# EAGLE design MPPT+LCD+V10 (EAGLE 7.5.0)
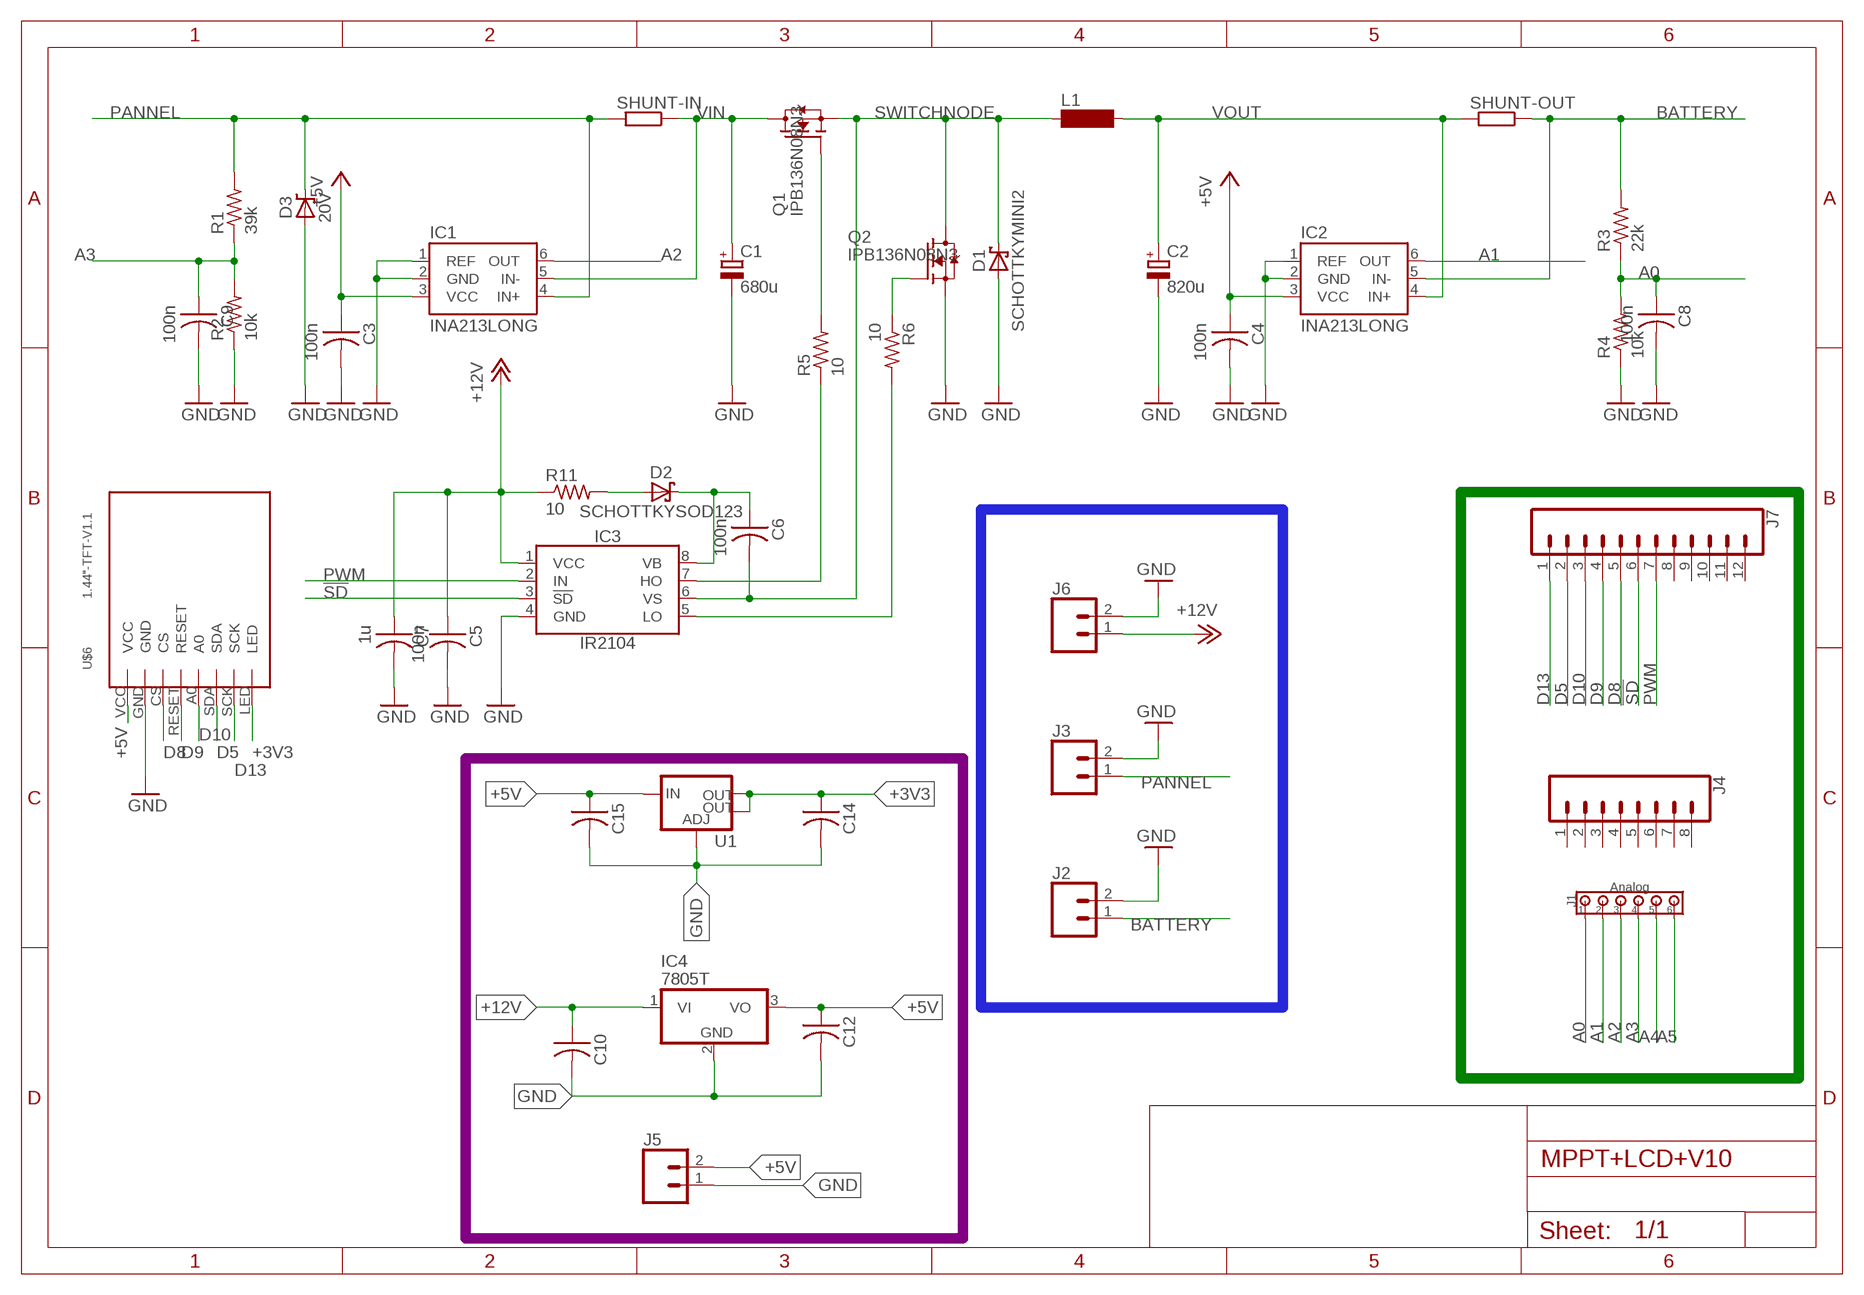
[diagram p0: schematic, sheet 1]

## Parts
C1  680u  C_POLARIZED10MM  [10MM]
C2  820u  C_POLARIZED10MM  [10MM]
C3  100n  CAP-US1206FAB  [C1206FAB]
C4  100n  CAP-US1206FAB  [C1206FAB]
C5  100n  CAP-US1206FAB  [C1206FAB]
C6  100n  CAP-US1206FAB  [C1206FAB]
C7  1u  CAP-US1206FAB  [C1206FAB]
C8  100n  CAP-US1206FAB  [C1206FAB]
C9  100n  CAP-US1206FAB  [C1206FAB]
C10  CAP-US1206FAB  [C1206FAB]
C12  CAP-US1206FAB  [C1206FAB]
C14  CAP-US1206FAB  [C1206FAB]
C15  CAP-US1206FAB  [C1206FAB]
D1  SCHOTTKYMINI2  [MINI2-F3-B]
D2  SCHOTTKYSOD123  [SOD123]
D3  20V  ZENERSMC  [SMC]
IC1  INA213LONG  [SC70-6_LONG]
IC2  INA213LONG  [SC70-6_LONG]
IC3  IR2104  [SOIC8]
IC4  7805T  [TO220H]
J1  Analog  100MIL_6X  [100MIL_6X_ROUND]
J2  CONN_02PTH4  [1X02_XTRA_BIG]
J3  CONN_02PTH4  [1X02_XTRA_BIG]
J4  CONN_08"  [1X08]
J5  CONN_02  [1X02]
J6  CONN_02PTH4  [1X02_XTRA_BIG]
J7  CONN_12  [1X12]
L1  SD75  [SD75]
Q1  IPB136N08N3  N-PWR-MOSFETTO263-3  [TO263-3]
Q2  IPB136N08N3  IPB136N08N3_GTO263  [TO263-3@1]
R1  39k  RES-US1206FAB  [R1206FAB]
R2  10k  RES-US1206FAB  [R1206FAB]
R3  22k  RES-US1206FAB  [R1206FAB]
R4  10k  RES-US1206FAB  [R1206FAB]
R5  10  RES-US1206FAB  [R1206FAB]
R6  10  RES-US1206FAB  [R1206FAB]
R11  10  RES-US1206FAB  [R1206FAB]
SHUNT-IN  SMR  [SMR]
SHUNT-OUT  SMR  [SMR]
U1  V_REG_LM1117SOT223  [SOT223]
U$6  1.44"-TFT-V1.1  [1.44-TFT-V1.1]

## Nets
!SD!: IC3.3(!SD!) J7.6
+3V3: C14.1 U1.2(OUT) U1.4(OUT) U$6.LED
+5V: C3.1 C4.1 C12.1 C15.1 IC1.3(VCC) IC2.3(VCC) IC4.3(VO) J5.2 U1.3(IN) U$6.VCC
+12V: C5.1 C7.1 C10.1 IC3.1(VCC) IC4.1(VI) J6.1 R11.1
A0: C8.1 J1.1 R3.1 R4.2
A1: IC2.6(OUT) J1.2
A2: IC1.6(OUT) J1.3
A3: C9.1 J1.4 R1.1 R2.2
A4: J1.5
A5: J1.6
BATTERY: IC2.5(IN-) J2.1 R3.2 SHUNT-OUT.1
D5: J7.2 U$6.SDA
D8: J7.5 U$6.CS
D9: J7.4 U$6.RESET
D10: J7.3 U$6.A0
D13: J7.1 U$6.SCK
GND: C1.- C2.- C3.2 C4.2 C5.2 C7.2 C8.2 C9.2 C10.2 C12.2 C14.2 C15.2 D1.A D3.A IC1.1(REF) IC1.2(GND) IC2.1(REF) IC2.2(GND) IC3.4(GND) IC4.2(GND) J2.2 J3.2 J5.1 J6.2 Q2.3(S) R2.1 R4.1 U1.1(ADJ) U$6.GND
N$4: Q1.1(G) R5.2
N$7: Q2.1(G) R6.1
N$11: D2.A R11.2
N$12: C6.1 D2.C IC3.8(VB)
N$14: IC3.7(HO) R5.1
N$15: IC3.5(LO) R6.2
PANNEL: D3.C IC1.4(IN+) J3.1 R1.2 SHUNT-IN.2
PWM: IC3.2(IN) J7.7
SWITCHNODE: C6.2 D1.C IC3.6(VS) L1.1 Q1.3(S) Q2.TAB(D)
VIN: C1.+ IC1.5(IN-) Q1.TAB(D) SHUNT-IN.1
VOUT: C2.+ IC2.4(IN+) L1.2 SHUNT-OUT.2
Unconnected: J4.1 J4.2 J4.3 J4.4 J4.5 J4.6 J4.7 J4.8 J7.8 J7.9 J7.10 J7.11 J7.12

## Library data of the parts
C1 C2 = 00Capacitor:C_POLARIZED
C3-C10 C12 C14 C15 = fab:CAP-US
D1 D2 = 00Diode:SCHOTTKY
D3 = 00Diode:ZENER
IC1 IC2 = 00Sensor:INA21*: Current-Shunt Monitors Voltage Output, Low- or High-Side Measurement, Bidirectional, Zero-Drift Series; GAIN: 50
IC3 = 00Logic:IR2104: Half-Bridge Driver Up to +600V Gate drive supply 10-20V Deadtime 520ns
IC4 = linear:78*: Positive VOLTAGE REGULATOR Source: http://cache.national.com/ds/LM/LM78L05.pdf http://www.fairchildsemi.com/ds/LM/LM7805.pdf
J1 = 00Connector:100MIL_6X: 100 mil 6-pin connector
J2 J3 J5 J6 = SparkFun-Connectors:CONN_02: Multi connection point. Often used as Generic Header-pin footprint for 0.1 inch spaced/style header connections
J4 = SparkFun-Connectors:CONN_08: Multi connection point. Often used as Generic Header-pin footprint for 0.1 inch spaced/style header connections On any of the 0.1 inch spaced packages, you can populate with these: Break Away Headers - Straight (PRT-00116) Break Away Male Headers - Right Angle (PRT-00553) Female Headers (PRT-00115)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; PROD_ID: CONN-08438
J7 = SparkFun-Connectors:CONN_12: Multi connection point. Often used as Generic Header-pin footprint for 0.1 inch spaced/style header connections On any of the 0.1 inch spaced packages, you can populate with these: Break Away Headers - Straight (PRT-00116) Break Away Male Headers - Right Angle (PRT-00553) Female Headers (PRT-00115)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
L1 = inductor-neosid:SD75: INDUCTOR; OC_FARNELL: unknown; OC_NEWARK: unknown
Q1 = 00Mosfet:N-PWR-MOSFET
Q2 = 00Mosfet:IPB136N08N3_G
R1-R6 R11 = fab:RES-US: Resistor (US Symbol)
SHUNT-IN SHUNT-OUT = resistor-shunt:SMR: SMD SHUNT RESISTOR; OC_FARNELL: unknown; OC_NEWARK: unknown
U1 = fab:V_REG_LM1117: Voltage Regulator LM1117 Standard adjustable voltage regulator but in SMD form. Spark Fun Electronics SKU : COM-00595; PROD_ID: VREG-08170
U$6 = tft_1.8_1.44_oled_0.96:1.44"-TFT-V1.1

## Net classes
0 default: clearance 0.205 mm

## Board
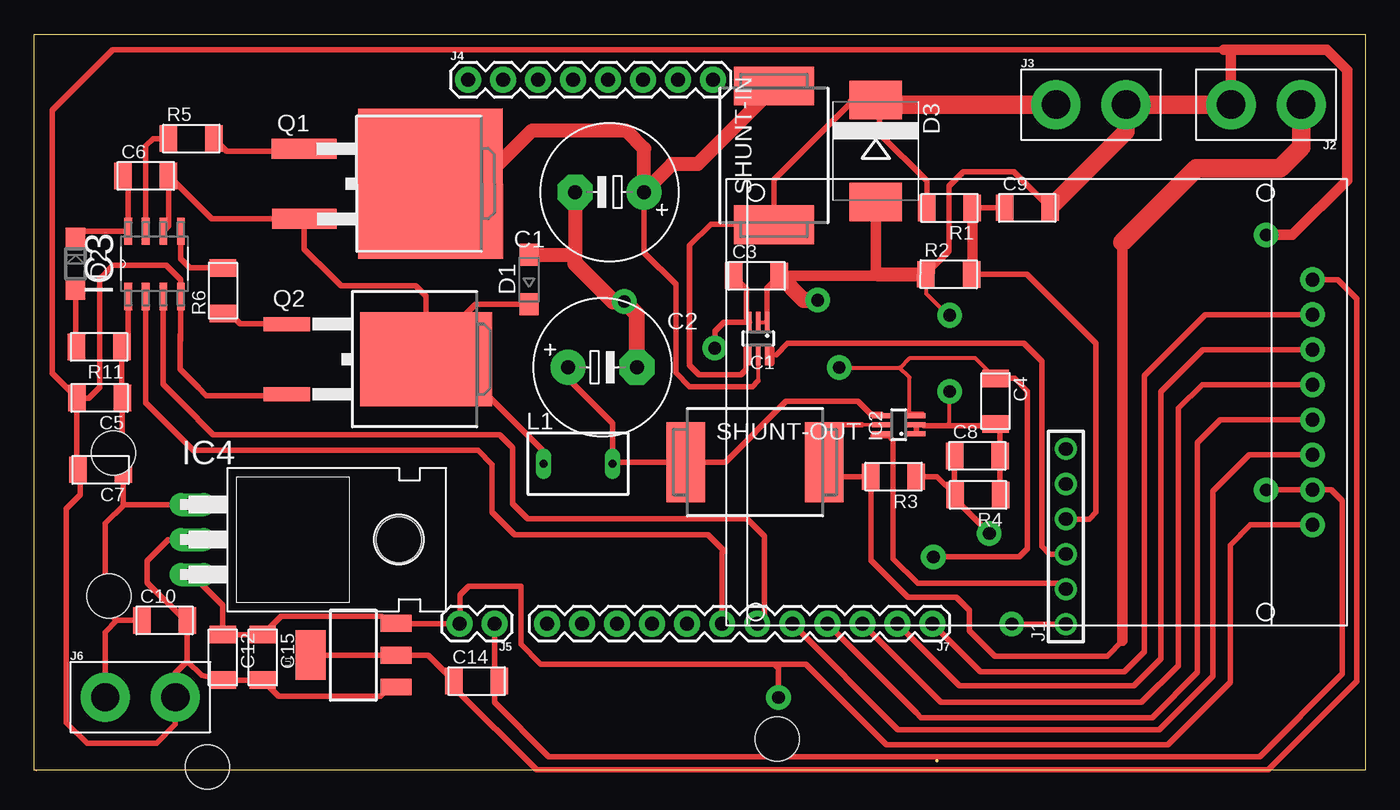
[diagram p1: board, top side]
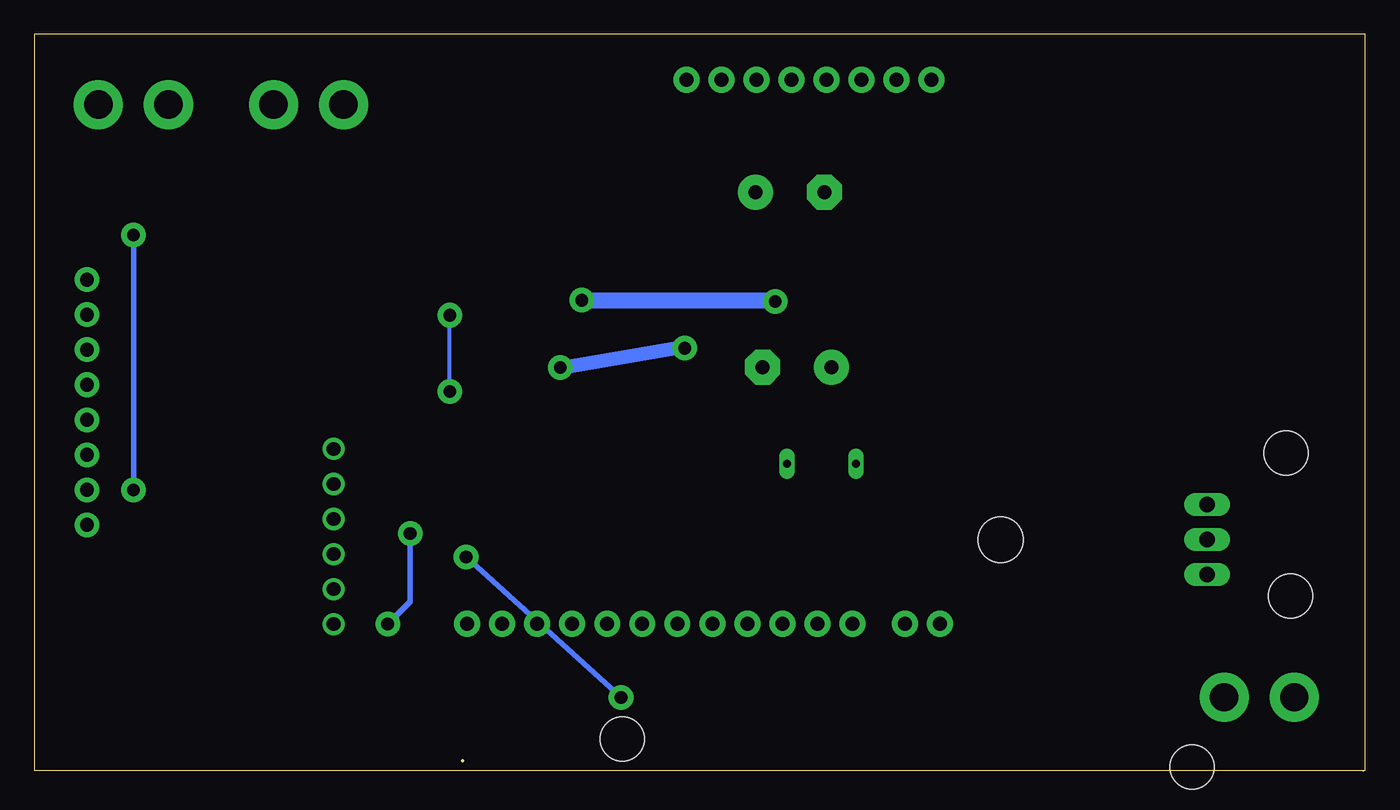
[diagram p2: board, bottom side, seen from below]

Size 96.52 x 53.42 mm. Coordinates in mm from the lower left corner, seen from the top.
Outline: 65.46,0.75 arc-90 65.48,0.75
Outline: 0.15,0 0,0.08
Outline: 0,0.08 0,53.42 96.52,53.42 96.52,0.08 0,0.08
Copper layers (1*16): Top 0.035mm / dielectric 1.5mm / Bottom 0.035mm
Design rules "default *": minimum track width 10mil, minimum drill 24mil, track to track 12mil, track to pad 12mil, pad to pad 12mil, via to via 12mil, smd to smd 12mil, copper to edge 0mil, drill to drill 8mil, minimum pad ring 10mil, minimum via ring 8mil, stop-mask expansion 4mil, vias tented up to drill 0mil, thermal gap 10mil
Holes 3.2 mm at 5.72,23.05 53.86,2.33 5.39,12.71 12.56,0.3

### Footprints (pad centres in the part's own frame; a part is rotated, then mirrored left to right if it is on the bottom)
10MM = drill 1.016 pad 2.54: + -2.5,0 | drill 1.016 pad 2.54 octagon: - 2.5,0
C1206FAB = smd 1.27 x 1.905: 1 -1.651,0; 2 1.651,0
MINI2-F3-B = smd 1.6 x 1.4: A 1.8,0; C -1.8,0
SOD123 = smd 1.4 x 1.4: A 1.9,0; C -1.9,0
SMC = smd 2.8 x 3.8: A 3.7,0; C -3.7,0
SC70-6_LONG = smd 0.35 x 1.5: 1 -0.65,-1.2; 2 0,-1.2; 3 0.65,-1.2; 4 0.65,1.2; 5 0,1.2; 6 -0.65,1.2
SOIC8 = smd 1.981 x 0.559: 1 -2.362,1.905; 2 -2.362,0.635; 3 -2.362,-0.635; 4 -2.362,-1.905; 5 2.362,-1.905; 6 2.362,-0.635; 7 2.362,0.635; 8 2.362,1.905
TO220H = drill 1.118 long: 1 -2.54,-10.16; 2 0,-10.16; 3 2.54,-10.16 | hole 3.302: 0,4.826
100MIL_6X_ROUND = drill 1 pad 1.6: 1 -6.35,0; 2 -3.81,0; 3 -1.27,0; 4 1.27,0; 5 3.81,0; 6 6.35,0
1X02_XTRA_BIG = drill 2.057 pad 3.556: 1 -2.54,0; 2 2.54,0
1X08 = drill 1.016 pad 1.88: 1 0,0; 2 2.54,0; 3 5.08,0; 4 7.62,0; 5 10.16,0; 6 12.7,0; 7 15.24,0; 8 17.78,0
1X02 = drill 1.016 pad 1.88: 1 0,0; 2 2.54,0
1X12 = drill 1.016 pad 1.88: 1 0,0; 2 2.54,0; 3 5.08,0; 4 7.62,0; 5 10.16,0; 6 12.7,0; 7 15.24,0; 8 17.78,0; 9 20.32,0; 10 22.86,0; 11 25.4,0; 12 27.94,0
SD75 = drill 0.6 long: 1 -2.5,0; 2 2.5,0
TO263-3 = smd 1.45 x 4.7: 1 -2.54,-5.65; 3 2.54,-5.65 | smd 10.9 x 10.5: TAB 0,3.5
TO263-3@1 = smd 1 x 3.4: 1 -2.54,-6.6; 3 2.54,-6.6 | smd 6.8 x 9.6: TAB 0,3.5
R1206FAB = smd 1.27 x 1.905: 1 -1.651,0; 2 1.651,0
SMR = smd 2.8 x 5.8: 1 5.029,0; 2 -5.029,0
SOT223 = smd 1.219 x 2.235: 1 -2.311,-3.099; 2 0,-3.099; 3 2.311,-3.099 | smd 3.6 x 2.2: 4 0,3.099
1.44-TFT-V1.1 = drill 1 pad 1.778: A0 0,7.62; CS 0,12.7; GND 0,15.24; LED 0,0; RESET 0,10.16; SCK 0,2.54; SDA 0,5.08; VCC 0,17.78

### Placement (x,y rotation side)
C1  41.72,41.99 180 top
C2  41.19,29.29 0 top
C3  52.38,35.92 0 top
C4  69.72,26.83 270 top
C5  4.73,27.07 180 top
C6  8.08,43.16 0 top
C7  4.79,21.85 180 top
C8  68.4,22.85 0 top
C9  72.01,40.85 0 top
C10  9.43,10.93 0 top
C12  13.66,8.26 270 top
C14  32.09,6.53 0 top
C15  16.56,8.25 270 top
D1  35.88,35.64 90 top
D2  2.98,36.79 270 top
D3  61.03,44.97 270 top
IC1  52.5,31.37 180 top
IC2  62.69,25.12 90 top
IC3  8.71,36.79 90 top
IC4  21.61,16.79 270 top
J1  74.82,17.01 90 top
J2  89.34,48.34 180 top
J3  76.64,48.34 0 top
J4  31.44,50.14 0 top
J5  33.38,10.7 180 top
J6  7.68,5.36 0 top
J7  65.13,10.7 180 top
L1  39.43,22.29 0 top
Q1  25.23,42.59 270.1 top
Q2  24.91,29.87 270 top
R1  66.37,40.84 180 top
R2  66.32,36.03 359.7 top
R3  62.32,21.36 180 top
R4  68.45,20.03 180 top
R5  11.38,45.87 0 top
R6  13.68,34.85 90 top
R11  4.69,30.76 180 top
SHUNT-IN  53.65,44.65 90 top
SHUNT-OUT  52.27,22.41 0 top
U1  23.13,8.41 90 top
U$6  92.71,35.64 180 top

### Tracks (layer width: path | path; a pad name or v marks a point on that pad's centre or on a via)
!SD!
  Top 0.406: IC3.3 9.35,28.06 11.83,25.57 11.83,25.53 12.98,24.38 33.74,24.38 34.67,23.45 34.67,19.4 35.76,18.31 51.68,18.31 52.96,17.03 52.96,11.23 J7.6
+3V3
  Top 0.406: U1.4 U1.2 28.55,8.41 C14.1 30.44,6.06 36.41,0.09 89.5,0.09 95.92,6.51 95.92,34.25 94.53,35.64 U$6.LED
+5V  (via drill 0.91 pad 1.78)
  Top 0.254: IC1.3 51.66,32.57 51.65,32.56
  Top 0.305: IC2.3 63.65,25.77 63.47,25.95 | 63.47,25.95 64.42,25.95 | v58.37,29.26 62.76,29.26 | 62.76,29.26 62.8,29.26 63.51,29.97 68.23,29.97 C4.1 | 63.47,25.95 63.47,28.55 62.76,29.26
  Top 0.406: IC4.3 13.66,12.04 C12.1 13.67,9.9 C15.1 17.88,11.22 25.17,11.22 25.66,10.72 U1.3 26.25,10.7 J5.2 30.88,10.74 30.88,12.8 31.48,13.4 35.29,13.4 35.29,9.2 36.72,7.77 53.67,7.77 | 51.65,32.56 51.65,34.99 C3.1 | 53.67,7.77 55.96,7.77 61.8,1.93 82.23,1.93 86.73,6.43 86.73,16.38 88.21,17.86 U$6.VCC | IC1.3 50.02,32.57 49.36,31.91 v49.36,30.67 | C4.1 71.12,28.48 72.04,27.56 72.04,16.12 71.79,15.87 71.49,15.57 71.45,15.53 v65.21,15.53 | v53.97,5.35 53.97,7.47 53.67,7.77
  Bottom 0.406: v65.21,15.53 v53.97,5.35
  Bottom 1.016: v58.37,29.26 49.46,30.77 v49.36,30.67
+12V
  Top 0.406: IC3.1 6.81,31.23 R11.1 6.34,27.11 C5.1 6.38,21.92 C7.1 6.44,19.44 6.42,19.42 6.5,19.33 | C10.1 5.98,10.93 | 5.98,10.93 5.14,11.77 5.14,17.96 6.5,19.33 | J6.1 5.14,10.09 5.98,10.93 | IC4.1 6.5,19.33
A0  (via drill 0.91 pad 1.78)
  Top 0.406: C8.1 66.75,20.08 R4.2 | R3.1 65.47,21.36 R4.2 | R4.2 66.79,19.72 v69.27,17.24 | v70.9,10.67 J1.1
  Bottom 0.406: v69.27,17.24 69.27,12.3 v70.9,10.67
A1
  Top 0.254: IC2.6 60.99,24.47 60.83,24.31
  Top 0.406: 60.83,24.31 61.97,24.31 62.29,23.99 62.29,15.39 64.07,13.61 74.27,13.61 74.68,13.2 J1.2
A2
  Top 0.254: IC1.6 53.15,30.34
  Top 0.305: 53.44,30.66 53.15,30.37 IC1.6 53.17,30.19 53.81,30.19
  Top 0.406: J1.3 73.64,15.74 73.08,16.3 73.08,29.72 71.78,31.02 54.64,31.02 53.81,30.19
  Top 0.508: 53.44,30.66 53.44,29.61
A3
  Top 0.406: R1.1 70.36,40.84 C9.1 | R2.2 72,36.02 76.98,31.04 76.98,18.76 76.5,18.28 J1.4
  Top 0.762: R1.1 68.02,36.07 R2.2
BATTERY
  Top 0.254: IC2.5 60.02,25.12
  Top 0.305: 57.91,24.79 57.07,23.96 57.07,23.16 57.31,22.92 57.31,22.42 SHUNT-OUT.1
  Top 0.406: SHUNT-OUT.1 58.35,21.36 R3.2 60.67,15.29 63.35,12.61 66.86,12.61 67.81,11.66 67.81,10.19 69.67,8.33 77.81,8.33 78.92,9.44 | 60.02,25.12 58.23,25.12 57.91,24.79
  Top 0.762: 78.92,38.37 78.92,9.44
  Top 1.346: J2.1 91.88,45.25 90.36,43.73 84.28,43.73 78.92,38.37
D5
  Top 0.406: J7.2 66.7,6.59 66.83,6.46 67.1,6.19 79.76,6.19 81.72,8.15 81.72,27.51 84.77,30.56 U$6.SDA
D8
  Top 0.406: J7.5 62.65,3.02 81.61,3.02 85.48,6.89 85.48,20.29 88.13,22.94 U$6.CS
D9
  Top 0.406: J7.4 63.73,4.48 63.99,4.22 64.32,3.89 81.1,3.89 84.37,7.16 84.37,23.83 86.02,25.48 U$6.RESET
D10
  Top 0.406: J7.3 65.76,4.99 80.31,4.99 82.98,7.66 82.98,26.3 84.7,28.02 U$6.A0
D13
  Top 0.406: J7.1 68.62,7.21 79.06,7.21 80.52,8.67 80.52,28.69 84.93,33.1 U$6.SCK
GND  (via drill 0.91 pad 1.78)
  Top 0.254: 64.53,25.05 64.46,25.12 IC2.2 63.93,25.12 63.99,25.06
  Top 0.305: IC1.2 IC1.1 | 64.46,25.12 66.25,25.12 66.37,25.24 66.37,27.51 v66.39,27.53 | v66.39,33.06 66.26,33.06 64.67,34.65 R2.1
  Top 0.406: 10.61,31.23 10.61,31.66 | 10.61,31.66 10.61,34.42 | 10.61,34.42 IC3.4 | 10.61,34.42 10.61,35.62 9.54,36.68 5.69,36.68 4.72,35.71 4.72,27.84 3.93,27.05 3.09,27.05 C5.2 | C5.2 3.08,21.92 C7.2 3.26,21.85 3.33,21.92 3.33,20.04 2.31,19.03 2.31,3.53 3.81,2.03 8.85,2.03 10.22,3.39 J6.2 10.22,7.1 11.09,7.97 | 54.04,35.91 C3.2 53.15,35.04 IC1.1 | R4.1 70.05,20.08 C8.2 70.05,24.85 C4.2 69.59,25.05 64.53,25.05 | 10.61,31.66 10.59,31.64 10.59,29.13 11.92,27.8 11.92,27.79 12.47,27.24 18.22,27.24 Q2.3 | IC4.2 9.71,16.79 8.17,15.26 8.17,13.68 10.92,10.93 C10.2 11.09,7.97 | C12.2 12.12,6.94 11.09,7.97 | C12.2 13.66,6.2 | 63.99,25.06 63.99,24.57 IC2.1 | C12.2 13.67,6.59 C15.2 17.71,5.44 25.12,5.44 25.78,6.1 U1.1 26.52,6.39 | J5.1 33.38,6.89 | 33.38,6.89 C14.2 | v89.35,20.38 89.37,20.4 U$6.GND 94.08,20.4 94.88,19.6 94.88,7.05 88.89,1.06 37.31,1.06 33.38,4.99 33.38,6.89 | 86.77,52.31 86.28,52.31 5.69,52.31 1.29,47.91 1.29,28.85 C5.2 | C9.2 71.03,43.48 67.39,43.48 66.33,42.42 66.33,37.7 R2.1
  Top 0.762: J2.2 86.8,52.28 86.77,52.31 | 86.28,52.31 93.75,52.31 95.22,50.84 95.22,42.86 91.25,38.89 v89.33,38.89 | C3.2 60.87,35.92 61.03,36.08 | D3.A 61.03,36.08 | 61.07,36.04 61.03,36.08
  Top 1.016: C1.- 39.22,37.18 | 39.22,37.18 39.22,36.83 | D1.A 38.96,37.44 39.22,37.18 | 61.07,36.04 R2.1
  Top 1.168: C2.- 43.69,33.14 v42.77,34.06 41.99,34.06 39.22,36.83 | v56.82,34.15 55.8,34.15 C3.2
  Top 1.27: 79.18,47.44 79.18,46.36 C9.2
  Top 1.346: 79.18,47.44 J3.2 J2.2
  Bottom 0.305: v66.39,27.53 v66.39,33.06
  Bottom 0.406: v89.33,38.89 89.33,20.4 v89.35,20.38
  Bottom 1.168: v56.82,34.15 42.87,34.15 v42.77,34.06
N$4
  Top 0.406: Q1.1 19.4,44.95 13.96,44.95 R5.2
N$7
  Top 0.406: 13.95,33.34 13.81,33.2 R6.1 14.15,33.2 14.91,32.44 18.28,32.44 Q2.1
N$11
  Top 0.406: D2.A 2.98,30.82 R11.2
N$12
  Top 0.406: C6.1 6.81,42.78 IC3.8 3.44,39.15 D2.C
N$14
  Top 0.406: IC3.7 8.08,45.35 8.6,45.87 R5.1
N$15
  Top 0.406: IC3.5 10.62,37.14 11.26,36.5 R6.2
PANNEL
  Top 0.254: IC1.4 51.85,30.45 51.62,30.68
  Top 0.406: 51.62,30.68 51.62,29.12 51.24,28.74 48.21,28.74 47.53,29.42 47.53,38.13 49.07,39.67 53.6,39.67 SHUNT-IN.2 53.65,42.89 59.35,48.59 59.22,48.59 59.19,48.62 60.58,48.62 D3.C 60.76,48.4 60.76,47.93 60.95,47.74 61.11,47.74 61.3,47.55 61.3,46.23 64.72,42.81 R1.2
  Top 1.346: J3.1 61.36,48.34 D3.C
PWM
  Top 0.406: IC3.2 8.08,26.71 11.52,23.26 32.17,23.26 33.2,22.23 33.2,18.76 34.81,17.15 48.85,17.15 49.94,16.06 49.94,15.87 49.89,15.82 J7.7
SWITCHNODE
  Top 0.406: 28.41,30.35 Q2.TAB 28.4,29.88 28.4,30.52 | IC3.6 9.73,39.53 C6.2 12.84,40.05 Q1.3 19.58,37.86 21.57,35.86 21.94,35.5 22.25,35.19 27.64,35.19 28.4,34.43 28.4,30.52 | 28.66,30.52 29.61,30.52 36.93,23.2 L1.1 | 28.66,30.52 28.4,30.52 | D1.C 31.98,33.84 28.66,30.52
VIN
  Top 0.305: IC1.5 52.5,28.3
  Top 0.406: 52.5,28.3 52.08,27.88 47.53,27.88 46.52,28.89 46.52,35.29 44.22,37.59 C1.+ | SHUNT-IN.1 53.63,49.66 53.63,49.54
  Top 1.016: Q1.TAB 32.23,42.6 36.1,46.47 42.9,46.47 44.22,45.15 C1.+ 46.24,44.01 48.1,44.01 53.63,49.54
VOUT
  Top 0.254: IC2.4 61.49,25.84 61.44,25.89
  Top 0.406: 61.44,25.89 60.67,25.89 59.74,26.82 54.53,26.82 50.12,22.41 SHUNT-OUT.2 42.05,22.41 L1.2 41.93,25.23 38.69,28.47 C2.+

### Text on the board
tText: Pan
